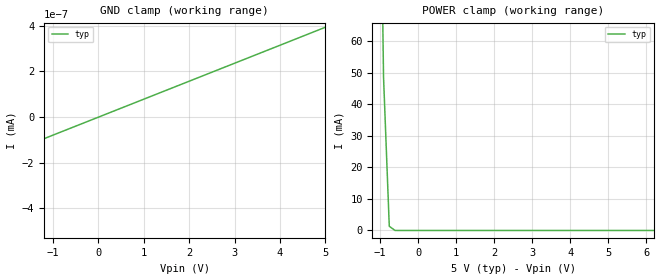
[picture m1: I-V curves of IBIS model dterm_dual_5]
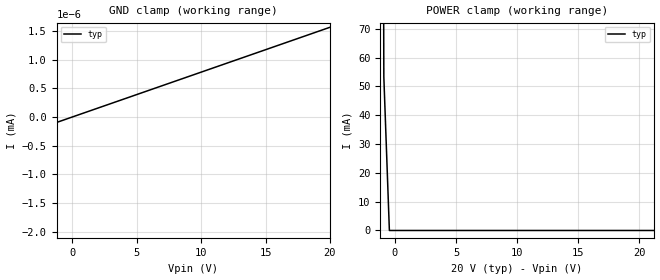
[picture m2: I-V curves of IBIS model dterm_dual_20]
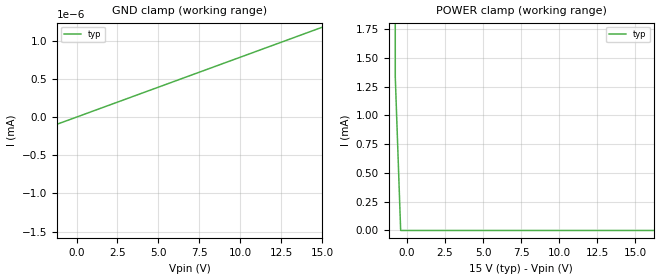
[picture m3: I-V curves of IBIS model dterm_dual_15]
|Texas Instruments Incorporated
|tmux7201, 1 Data Lane 1:1 44V Precision mux
[IBIS Ver]   4.1
[File name]   tmux7201.ibs
[Date]   12/01/22
[File Rev]   1.0
[Source]
| Texas Instruments Incorporated.
| ASC-INT-MPD
| 12500 TI Blvd
| Dallas, TX - 75243
[Notes]   Revision History:
| Rev 1.0: 12/01/22
| - Initial version of the model
| - Model generated from simulations in SPECTRE
| - C_comp although listed in numerical order of value are
|   obtained from varying PVT conditions. For PVT conditions for
|   each specific value refer the buffer description under
|   respective [Model]. IBIS model user is responsible for using
|   appropriate C_comp to simulate for Signal Integrity.
[Disclaimer]
| This model is designed as an aid for customers of Texas Instruments.
| TI and its licensors and suppliers make no warranties, either expressed
| or implied, with respect to this  model, including the warranties of
| merchantability or fitness for a particular purpose. The model is
| provided solely on an "as is" basis. The entire risk as to its quality
| and performance is with the customer.
| This model is subject to change without notice. Texas Instruments
| Incorporated is not responsible for updating this model.
[Copyright]
(C) Copyright 2022 Texas Instruments Incorporated.All rights reserved.
|  Component TMUX7201DGK 8-pin - DGK package
|  Part # TMUX7201DGK
[Component]   TMUX7201DGK
[Manufacturer]  TI
[Package]
|   typ   min   max
R_pkg   0.0668   NA   NA
L_pkg   2.1992nH   NA   NA
C_pkg   0.2884pF   NA   NA
[Pin]   signal_name   model_name
   1   S   sterm
   2   NC   nc
   3   GND   gnd
   4   VDD   power
   5   NC   nc
   6   SEL   inbuf
   7   VSS   power
   8   D   dterm
[Series Switch Groups]
On 1 /
Off 1 /
[Series Pin Mapping]  pin_2 model_name function_table_group
   1   8   switch_dual_5   1
|   1   8   switch_dual_20   1
|   1   8   switch_dual_15   1
|   1   8   switch_36   1
|   1   8   switch_44   1
|   1   8   switch_12   1
|  Component TMUX7201RQX 8-pin - RQX package
|  Part # TMUX7201RQX
[Component]   TMUX7201RQX
[Manufacturer]  TI
[Package]
|   typ   min   max
R_pkg   0.0668   NA   NA
L_pkg   2.1992nH   NA   NA
C_pkg   0.2884pF   NA   NA
[Pin]   signal_name   model_name
   1   S   sterm
   2   NC   nc
   3   GND   gnd
   4   VDD   power
   5   NC   nc
   6   SEL   inbuf
   7   VSS   power
   8   D   dterm
[Series Switch Groups]
On 1 /
Off 1 /
[Series Pin Mapping]  pin_2 model_name function_table_group
|   1   8   switch_dual_5   1
|   1   8   switch_dual_20   1
|   1   8   switch_dual_15   1
|   1   8   switch_36   1
|   1   8   switch_44   1
   1   8   switch_12   1
[Model Selector] dterm
dterm_dual_5 Use for operation at +/-5V
dterm_dual_20 Use for operation at +/-20V
dterm_dual_15 Use for operation at +/-15V
dterm_36 Use for operation at 36V
dterm_44 Use for operation at 44V
dterm_12 Use for operation at 12V
[Model Selector] sterm
sterm_dual_5 Use for operation at +/-5V
sterm_dual_20 Use for operation at +/-20V
sterm_dual_15 Use for operation at +/-15V
sterm_36 Use for operation at 36V
sterm_44 Use for operation at 44V
sterm_12 Use for operation at 12V
[Model Selector] inbuf
inbuf_dual_5 Use for operation at +/-5V
inbuf_dual_20 Use for operation at +/-20V
inbuf_dual_15 Use for operation at +/-15V
inbuf_36 Use for operation at 36V
inbuf_44 Use for operation at 44V
inbuf_12 Use for operation at 12V
| switch_dual_5
[Model]   switch_dual_5
Model_type   Series_switch
|   typ   min   max
C_comp   2.533030e-11   NA   NA
[Voltage Range]   5   NA   NA
[Power Clamp Reference]   5   NA   NA
[Temperature Range]   27   NA   NA
[On]
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[Off]
|   typ   min   max
[R Series]   10G   NA   NA
| switch_dual_20
[Model]   switch_dual_20
Model_type   Series_switch
|   typ   min   max
C_comp   4.014581e-11   NA   NA
[Voltage Range]   20   NA   NA
[Power Clamp Reference]   20   NA   NA
[Temperature Range]   27   NA   NA
[On]
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[Off]
|   typ   min   max
[R Series]   10G   NA   NA
| switch_dual_15
[Model]   switch_dual_15
Model_type   Series_switch
|   typ   min   max
C_comp   4.014581e-11   NA   NA
[Voltage Range]   15   NA   NA
[Power Clamp Reference]   15   NA   NA
[Temperature Range]   27   NA   NA
[On]
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[Off]
|   typ   min   max
[R Series]   10G   NA   NA
| switch_36
[Model]   switch_36
Model_type   Series_switch
|   typ   min   max
C_comp   4.014581e-11   NA   NA
[Voltage Range]   36   NA   NA
[Power Clamp Reference]   36   NA   NA
[Temperature Range]   27   NA   NA
[On]
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[Off]
|   typ   min   max
[R Series]   10G   NA   NA
| switch_44
[Model]   switch_44
Model_type   Series_switch
|   typ   min   max
C_comp   4.014581e-11   NA   NA
[Voltage Range]   44   NA   NA
[Power Clamp Reference]   44   NA   NA
[Temperature Range]   27   NA   NA
[On]
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[Off]
|   typ   min   max
[R Series]   10G   NA   NA
| switch_12
[Model]   switch_12
Model_type   Series_switch
|   typ   min   max
C_comp   2.533030e-11   NA   NA
[Voltage Range]   12   NA   NA
[Power Clamp Reference]   12   NA   NA
[Temperature Range]   27   NA   NA
[On]
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[Off]
|   typ   min   max
[R Series]   10G   NA   NA
| Models and submodels in the file (24): dterm_dual_5 (Terminator), dterm_dual_20 (Terminator), dterm_dual_15 (Terminator), dterm_36 (Terminator), dterm_44 (Terminator), dterm_12 (Terminator), switch_dual_5 (Series_switch), switch_dual_20 (Series_switch), switch_dual_15 (Series_switch), switch_36 (Series_switch), switch_44 (Series_switch), switch_12 (Series_switch), sterm_dual_5 (Terminator), sterm_dual_20 (Terminator), sterm_dual_15 (Terminator), sterm_36 (Terminator), sterm_44 (Terminator), sterm_12 (Terminator), inbuf_dual_5 (Input), inbuf_dual_20 (Input), inbuf_dual_15 (Input), inbuf_36 (Input), inbuf_44 (Input), inbuf_12 (Input)
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| dterm_dual_5
[Model]   dterm_dual_5
Model_type   Terminator
|   typ   min   max
C_comp   2.533030e-11   NA   NA
[Voltage Range]   5   NA   NA
[Temperature Range]   27   NA   NA
[Power Clamp Reference]   5   NA   NA
[GND Clamp Reference]   0   NA   NA
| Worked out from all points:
|   GND clamp passes 1 mA (typ) near -5.72 V on its own axis
|   POWER clamp passes 1 mA (typ) near -0.72 V on its own axis
[GND Clamp]
|   Voltage   I(typ)   I(min)   I(max)
-10V      -11.28A    NA         NA
-5.303V   -789.5pA   NA         NA
-5.152V   -411pA     NA         NA
-5V       -394.1pA   NA         NA
5V        393.7pA    NA         NA
[POWER Clamp]
|   Voltage   I(typ)   I(min)   I(max)
-5V       13.24A     NA         NA
-1.061V   184.2mA    NA         NA
-909.1mV  48.72mA    NA         NA
-757.6mV  1.324mA    NA         NA
-606.1mV  6.572uA    NA         NA
10V       -394.1pA   NA         NA
| dterm_dual_20
[Model]   dterm_dual_20
Model_type   Terminator
|   typ   min   max
C_comp   4.014581e-11   NA   NA
[Voltage Range]   20   NA   NA
[Temperature Range]   27   NA   NA
[Power Clamp Reference]   20   NA   NA
[GND Clamp Reference]   0   NA   NA
[GND Clamp]
|   Voltage   I(typ)   I(min)   I(max)
-25V      -11.62A    NA         NA
-20.45V   -42.59nA   NA         NA
-20V      -1.566nA   NA         NA
20V       1.565nA    NA         NA
[POWER Clamp]
|   Voltage   I(typ)   I(min)   I(max)
-5V       13.27A     NA         NA
-1.364V   841.5mA    NA         NA
-909.1mV  53.34mA    NA         NA
-454.5mV  32.71nA    NA         NA
40V       -1.566nA   NA         NA
| dterm_dual_15
[Model]   dterm_dual_15
Model_type   Terminator
|   typ   min   max
C_comp   4.014581e-11   NA   NA
[Voltage Range]   15   NA   NA
[Temperature Range]   27   NA   NA
[Power Clamp Reference]   15   NA   NA
[GND Clamp Reference]   0   NA   NA
[GND Clamp]
|   Voltage   I(typ)   I(min)   I(max)
-20V      -11.55A    NA         NA
-15.4V    -9.308nA   NA         NA
-15.05V   -1.181nA   NA         NA
15V       1.176nA    NA         NA
[POWER Clamp]
|   Voltage   I(typ)   I(min)   I(max)
-5V       13.26A     NA         NA
-1.111V   275.7mA    NA         NA
-757.6mV  1.337mA    NA         NA
-404mV    6.544nA    NA         NA
30V       -1.177nA   NA         NA
